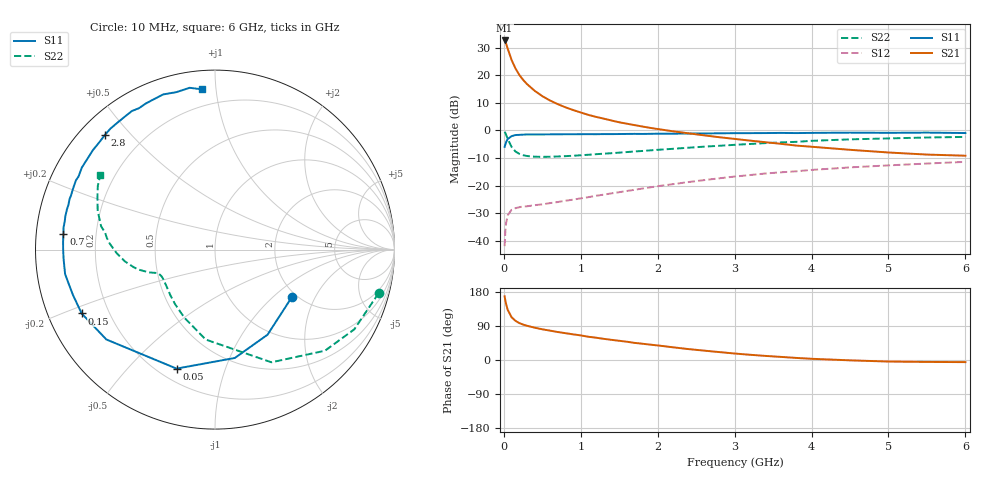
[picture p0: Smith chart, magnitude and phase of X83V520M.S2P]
! SIEMENS Small Signal Semiconductors
! BFP136W
! Si NPN RF Bipolar Junction Transistor in SOT343
! VCE = 3.5 V  IC = 20 mA
! Common Emitter S-Parameters:  September  1994
# GHz  S  MA  R  50
!  f  S11  S21  S12  S22
! GHz  MAG  ANG  MAG  ANG  MAG  ANG  MAG  ANG
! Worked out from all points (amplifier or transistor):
!   40 points, 10 MHz to 6 GHz, reference 50 ohm
!   highest |S21| = 32.6 dB at 10 MHz (marker M1)
!   |S21| within 3 dB of that: start of sweep to 50.53 MHz
!   unconditionally stable (mu >= 1): 875 MHz to 2.762 GHz
!   at 200 MHz: K = 0.33, MSG = 24.0 dB, |S12| = -27.8 dB
!   at 1.5 GHz: K = 1.16, MAG = 10.2 dB, |S12| = -22.4 dB
!   at 6 GHz: K = 0.98, MSG = 1.1 dB, |S12| = -11.4 dB
!   S11 on the Smith chart (normalised r, x): 10 MHz: 1.89, -1.33; 50 MHz: 0.27, -0.69; 150 MHz: 0.10, -0.22; 700 MHz: 0.08, +0.05; 2.8 GHz: 0.07, +0.42; 6 GHz: 0.10, +0.92
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0.01  0.5035 -31.6  42.58 168.2  0.008 77.5  0.9435 -14.9
0.02  0.5572 -58.3  39.84 156.9  0.0152 68.7  0.8941 -29.8
0.03  0.6138 -79.6  37.1 147.4  0.0211 59.6  0.8323 -42.6
0.05  0.6968 -107.9  30.29 132.5  0.029 46.1  0.7022 -63.4
0.1  0.7856 -140.4  18.97 113.0  0.0364 31.3  0.5038 -95.9
0.15  0.8237 -154.4  13.36 103.5  0.039 26.4  0.416 -114.2
0.2  0.8305 -162.1  10.17 97.6  0.0406 24.7  0.3768 -126.1
0.25  0.8379 -167.2  8.254 93.5  0.0419 24.2  0.3563 -134.1
0.3  0.8462 -170.8  6.925 90.4  0.0422 24.7  0.3438 -139.7
0.4  0.8452 -176.5  5.227 85.3  0.0442 26.7  0.3342 -146.9
0.5  0.8461 179.8  4.173 81.0  0.0458 29.0  0.3318 -151.4
0.6  0.8475 176.9  3.478 77.6  0.0482 31.7  0.3335 -153.9
0.7  0.8491 174.0  2.995 73.8  0.0504 34.7  0.3371 -155.5
0.9  0.8516 169.5  2.34 67.7  0.0557 38.9  0.3471 -157.9
1.1  0.855 164.8  1.908 61.3  0.0618 42.9  0.3623 -159.1
1.5  0.8597 157.6  1.404 50.7  0.076 48.7  0.3957 -161.6
2.2  0.8723 144.8  0.963 33.5  0.1063 51.6  0.4643 -167.9
2.8  0.8856 133.9  0.753 20.9  0.1356 50.0  0.5264 -175.3
3.2  0.892 127.3  0.653 13.8  0.1553 47.3  0.5673 179.3
4.5  0.9115 108.5  0.445 -0.9  0.2137 36.2  0.6881 161.8
5.5  0.9126 98.9  0.365 -5.1  0.2512 27.8  0.7435 151.4
6  0.8954 94.5  0.348 -5.6  0.2692 23.2  0.7624 147.0
